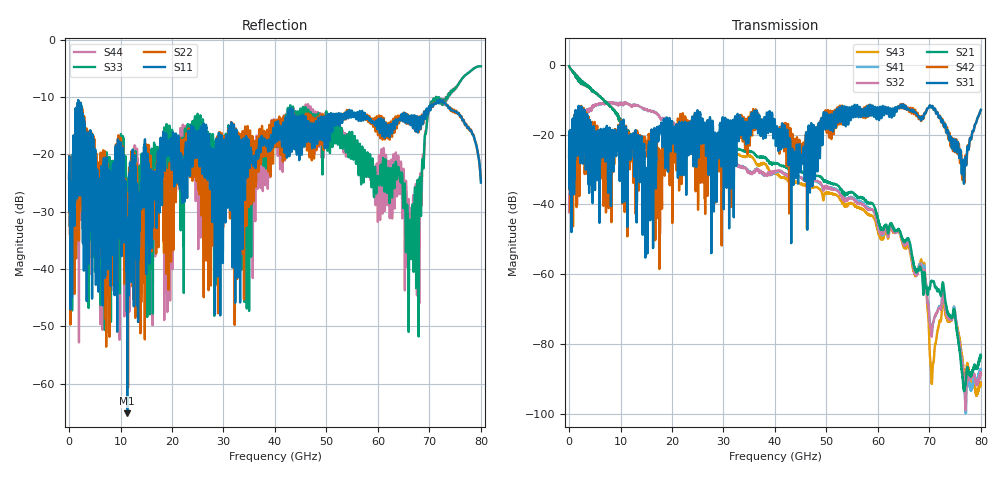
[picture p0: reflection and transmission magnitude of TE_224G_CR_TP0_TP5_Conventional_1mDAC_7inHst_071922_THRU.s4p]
!! Reference: tracy_3df_01a_2207
!! CHANNEL DESCRIPTION: TP0_TP5 CR Channel using 1meter DAC, Conventional 7in Host
!! MODEL DESCRIPTION: s4p, THRU
!! CONNECTOR DESCRIPTION: OSFP 200G SMT
!! CABLE DESCRIPTION: 1meter 26AWG Cable
!! MODEL STATUS: Developmental
!! PORT DEFINITIONS:
!! Port  1  ----->  Side A  Side B  <-----  Port  2
!! Port  3  ----->  Side A  Side B  <-----  Port  4
# GHz S MA R 50
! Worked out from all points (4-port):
!   8000 points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, 10 MHz to 80 GHz, reference 50 ohm
!   strongest paths, dB at 10 MHz, 20.01 GHz, 40.01 GHz, 60.01 GHz, 80 GHz:
!     S31: -26.6, -16.2, -17.4, -12.4, -12.9
!     S42: -26.6, -27.0, -18.6, -14.1, -13.0
!     S21: -0.5, -24.0, -28.2, -44.1, -83.5
!     S32: -42.2, -16.6, -30.6, -45.7, -88.5
!     S41: -42.2, -16.6, -30.7, -46.0, -87.7
!     S43: -0.5, -26.0, -31.1, -47.4, -91.6
!   lowest |S11| = -65.2 dB at 11.3 GHz (marker M1), VSWR 1.00, Z = 50 - j0.0496 ohm
!   |S11| at or under -10 dB: start of sweep to end of sweep
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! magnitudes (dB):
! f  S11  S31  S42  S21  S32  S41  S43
! 10 MHz  -24.3  -26.6  -26.6  -0.5  -42.2  -42.2  -0.5
! 11.3 GHz  -65.2  -29.0  -33.3  -18.7  -11.0  -11.0  -18.7
! 15.98 GHz  -29.0  -21.2  -19.9  -32.2  -13.4  -13.5  -36.3
! 46.19 GHz  -17.9  -24.3  -33.3  -31.4  -33.3  -33.2  -34.5
! 66.19 GHz  -14.0  -13.1  -13.1  -50.9  -52.4  -51.8  -53.3
! 70.37 GHz  -11.4  -12.3  -12.2  -62.0  -77.3  -76.5  -89.0
! 80 GHz  -24.9  -12.9  -13.0  -83.5  -88.5  -87.7  -91.6
